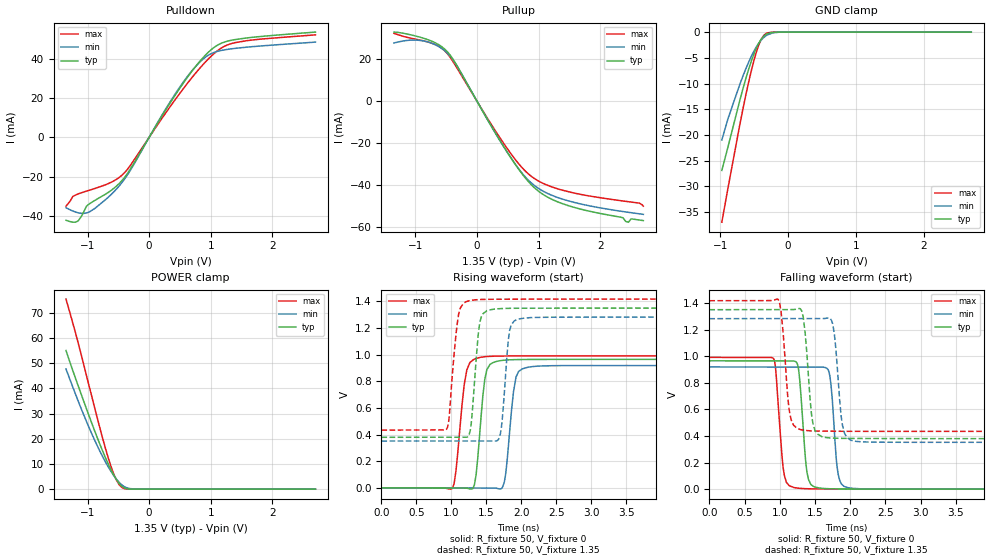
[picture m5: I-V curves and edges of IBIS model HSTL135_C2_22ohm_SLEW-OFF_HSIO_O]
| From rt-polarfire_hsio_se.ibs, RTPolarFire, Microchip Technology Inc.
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|   Model HSTL135_C2_22ohm_SLEW-OFF_HSIO_O
[Model]   HSTL135_C2_22ohm_SLEW-OFF_HSIO_O
Model_type   Output
Polarity   Non-Inverting
Enable   Active-High
Vmeas =   0.675
Cref =   5p
Rref =   50
Vref =   0.675
|   typ   min   max
C_comp_pullup   1.335e-12   1.335e-12   1.380e-12
C_comp_pulldown  1.335e-12   1.335e-12   1.380e-12
[Temperature Range]  25C   125C   -55C
[Voltage Range]  1.35   1.2825   1.4175
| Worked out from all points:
|   slope of the pulldown table from 0 to 0.203 V, typ, clamps not added: 19.1 ohm
|   slope of the pullup table from 0 to 0.203 V, typ, clamps not added: 19.5 ohm
|   GND clamp passes 1 mA (typ) near -0.37 V on its own axis
|   POWER clamp passes 1 mA (typ) near -0.43 V on its own axis
|   rising waveform, R_fixture 50, V_fixture 0: 20-80 % time 96.8ps typ, 99.7ps min, 111ps max; typ from 0 V to 0.966 V
|   rising waveform, R_fixture 50, V_fixture 1.35: 20-80 % time 85.4ps typ, 80.5ps min, 96.7ps max; typ from 0.38 V to 1.35 V
|   falling waveform, R_fixture 50, V_fixture 0: 20-80 % time 80.9ps typ, 74.9ps min, 83.5ps max; typ from 0.966 V to 0 V
|   falling waveform, R_fixture 50, V_fixture 1.35: 20-80 % time 85.3ps typ, 85.7ps min, 86.3ps max; typ from 1.35 V to 0.38 V
[GND Clamp]
| Voltage   I(typ)   I(min)   I(max)
-974.5mV  -26.9mA    -20.99mA   -36.97mA
-885.9mV  -22.43mA   -16.91mA   -30.47mA
-708.7mV  -13.23mA   -10.13mA   -17.94mA
-575.9mV  -7.072mA   -5.739mA   -9.511mA
-487.3mV  -3.767mA   -3.362mA   -4.833mA
-443mV    -2.466mA   -2.401mA   -2.954mA
-398.7mV  -1.449mA   -1.613mA   -1.504mA
-354.4mV  -738.4uA   -1.007mA   -579.6uA
-310.1mV  -318.4uA   -576.7uA   -161.6uA
-221.5mV  -38.75uA   -142.9uA   -7.637uA
-132.9mV  -3.522uA   -25.88uA   -362.7nA
2.7V      0A         0A         0A
[POWER Clamp]
| Voltage   I(typ)   I(min)   I(max)
-1.35V    55.07mA    47.72mA    75.49mA
-1.196V   44.05mA    37.75mA    62.13mA
-974.5mV  29.03mA    24.41mA    40.95mA
-797.3mV  17.68mA    14.97mA    24.06mA
-664.5mV  10.01mA    8.871mA    12.44mA
-575.9mV  5.63mA     5.451mA    6.064mA
-531.6mV  3.786mA    3.983mA    3.599mA
-487.3mV  2.262mA    2.712mA    1.789mA
-443mV    1.133mA    1.675mA    684.4uA
-354.4mV  127.5uA    473.3uA    30.46uA
-221.5mV  1.715uA    56.89uA    636.6nA
2.7V      0A         0A         0A
[Pullup]
| Voltage   I(typ)   I(min)   I(max)
-1.35V    33.08mA    27.87mA    32.5mA
-885.9mV  30.3mA     28.94mA    29mA
-487.3mV  23.84mA    23.19mA    22.97mA
-310.1mV  16.15mA    16.17mA    15.15mA
548.4mV   -26.94mA   -26.95mA   -24.98mA
801.6mV   -37.27mA   -36.73mA   -33.84mA
1.012V    -43.28mA   -41.9mA    -38.33mA
1.571V    -50.64mA   -48.26mA   -43.8mA
2.369V    -55.64mA   -52.66mA   -47.62mA
2.457V    -57.76mA   -53.04mA   -47.97mA
2.502V    -56.18mA   -53.22mA   -48.14mA
2.7V      -57mA      -54.01mA   -50.08mA
[Pulldown]
| Voltage   I(typ)   I(min)   I(max)
-1.35V    -42.21mA   -35.86mA   -35.04mA
-1.24V    -43.21mA   -37.52mA   -30.17mA
-1.152V   -42.55mA   -38.45mA   -28.81mA
-1.019V   -35.11mA   -38.55mA   -27.41mA
-575.9mV  -26.04mA   -27.86mA   -22.23mA
-354.4mV  -18.51mA   -19.22mA   -16.4mA
210.9mV   11.01mA    11.43mA    9.777mA
548.4mV   27.31mA    27.85mA    24.5mA
843.8mV   39.43mA    38.95mA    35.95mA
1.055V    45.79mA    43.23mA    42.67mA
1.394V    49.76mA    45.28mA    48.2mA
2.7V      53.58mA    48.48mA    52.17mA
[Ramp]
dV/dt_r   0.579308/96.7533p  0.551552/99.6539p  0.594875/0.111016n
dV/dt_f   0.582031/85.2881p  0.558376/85.6751p  0.58998/86.3381p
R_load = 50
[Rising Waveform]
R_fixture = 50
V_fixture = 0
V_fixture_min = 0
V_fixture_max = 0
| Time   V(typ)   V(min)   V(max)
0s        1.367uV    2.099uV    1.928uV
1.015ns   -724.7uV   -403.9uV   -2.773mV
1.219ns   -1.582mV   -485.5uV   884.3mV
1.328ns   21.65mV    -529.1uV   966.3mV
1.411ns   453.1mV    -562.3uV   979.9mV
1.506ns   887.7mV    -600.3uV   986.1mV
1.725ns   956.9mV    -268.4uV   989.8mV
1.923ns   963mV      832.7mV    990.2mV
2.092ns   964mV      905.8mV    990.4mV
10ns      965.5mV    919.3mV    991.5mV
[Rising Waveform]
R_fixture = 50
V_fixture = 1.35
V_fixture_min = 1.2825
V_fixture_max = 1.4175
| Time   V(typ)   V(min)   V(max)
0s        379.9mV    351.8mV    434.2mV
933ps     380.4mV    352.1mV    443.2mV
1.105ns   380.5mV    352.1mV    1.31V
1.258ns   410.2mV    352.2mV    1.405V
1.403ns   1.236V     352.2mV    1.414V
1.551ns   1.336V     352.2mV    1.416V
1.69ns    1.345V     386.1mV    1.416V
1.831ns   1.348V     1.182V     1.416V
1.994ns   1.349V     1.271V     1.417V
10ns      1.35V      1.282V     1.417V
[Falling Waveform]
R_fixture = 50
V_fixture = 0
V_fixture_min = 0
V_fixture_max = 0
| Time   V(typ)   V(min)   V(max)
0s        965.5mV    919.3mV    991.5mV
914ps     964.8mV    918.7mV    979.3mV
1.064ns   964.7mV    918.6mV    104.6mV
1.205ns   963.1mV    918.5mV    11.73mV
1.384ns   133.4mV    918.4mV    3.392mV
1.559ns   8.8mV      918.3mV    1.672mV
1.7ns     3.273mV    878.5mV    1.166mV
1.829ns   1.897mV    112mV      954.5uV
1.977ns   1.338mV    9.919mV    811.8uV
10ns      2.053uV    2.985uV    2.386uV
[Falling Waveform]
R_fixture = 50
V_fixture = 1.35
V_fixture_min = 1.2825
V_fixture_max = 1.4175
| Time   V(typ)   V(min)   V(max)
0s        1.35V      1.282V     1.417V
976ps     1.351V     1.283V     1.428V
1.133ns   1.351V     1.283V     596.6mV
1.307ns   1.345V     1.283V     446.9mV
1.469ns   498.8mV    1.283V     438.1mV
1.649ns   389.1mV    1.285V     436.4mV
1.775ns   383.6mV    1.167V     435.9mV
1.89ns    382.3mV    480.2mV    435.5mV
2.083ns   381.5mV    359.4mV    435.1mV
10ns      379.9mV    351.8mV    434.2mV
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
